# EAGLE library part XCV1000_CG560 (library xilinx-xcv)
xcv1000_cg560_1532 edit this description Auto generated by make-symbol-device-package-bsdl.ulp Rev. 26 Source: xcv1000_cg560_1532.bsd
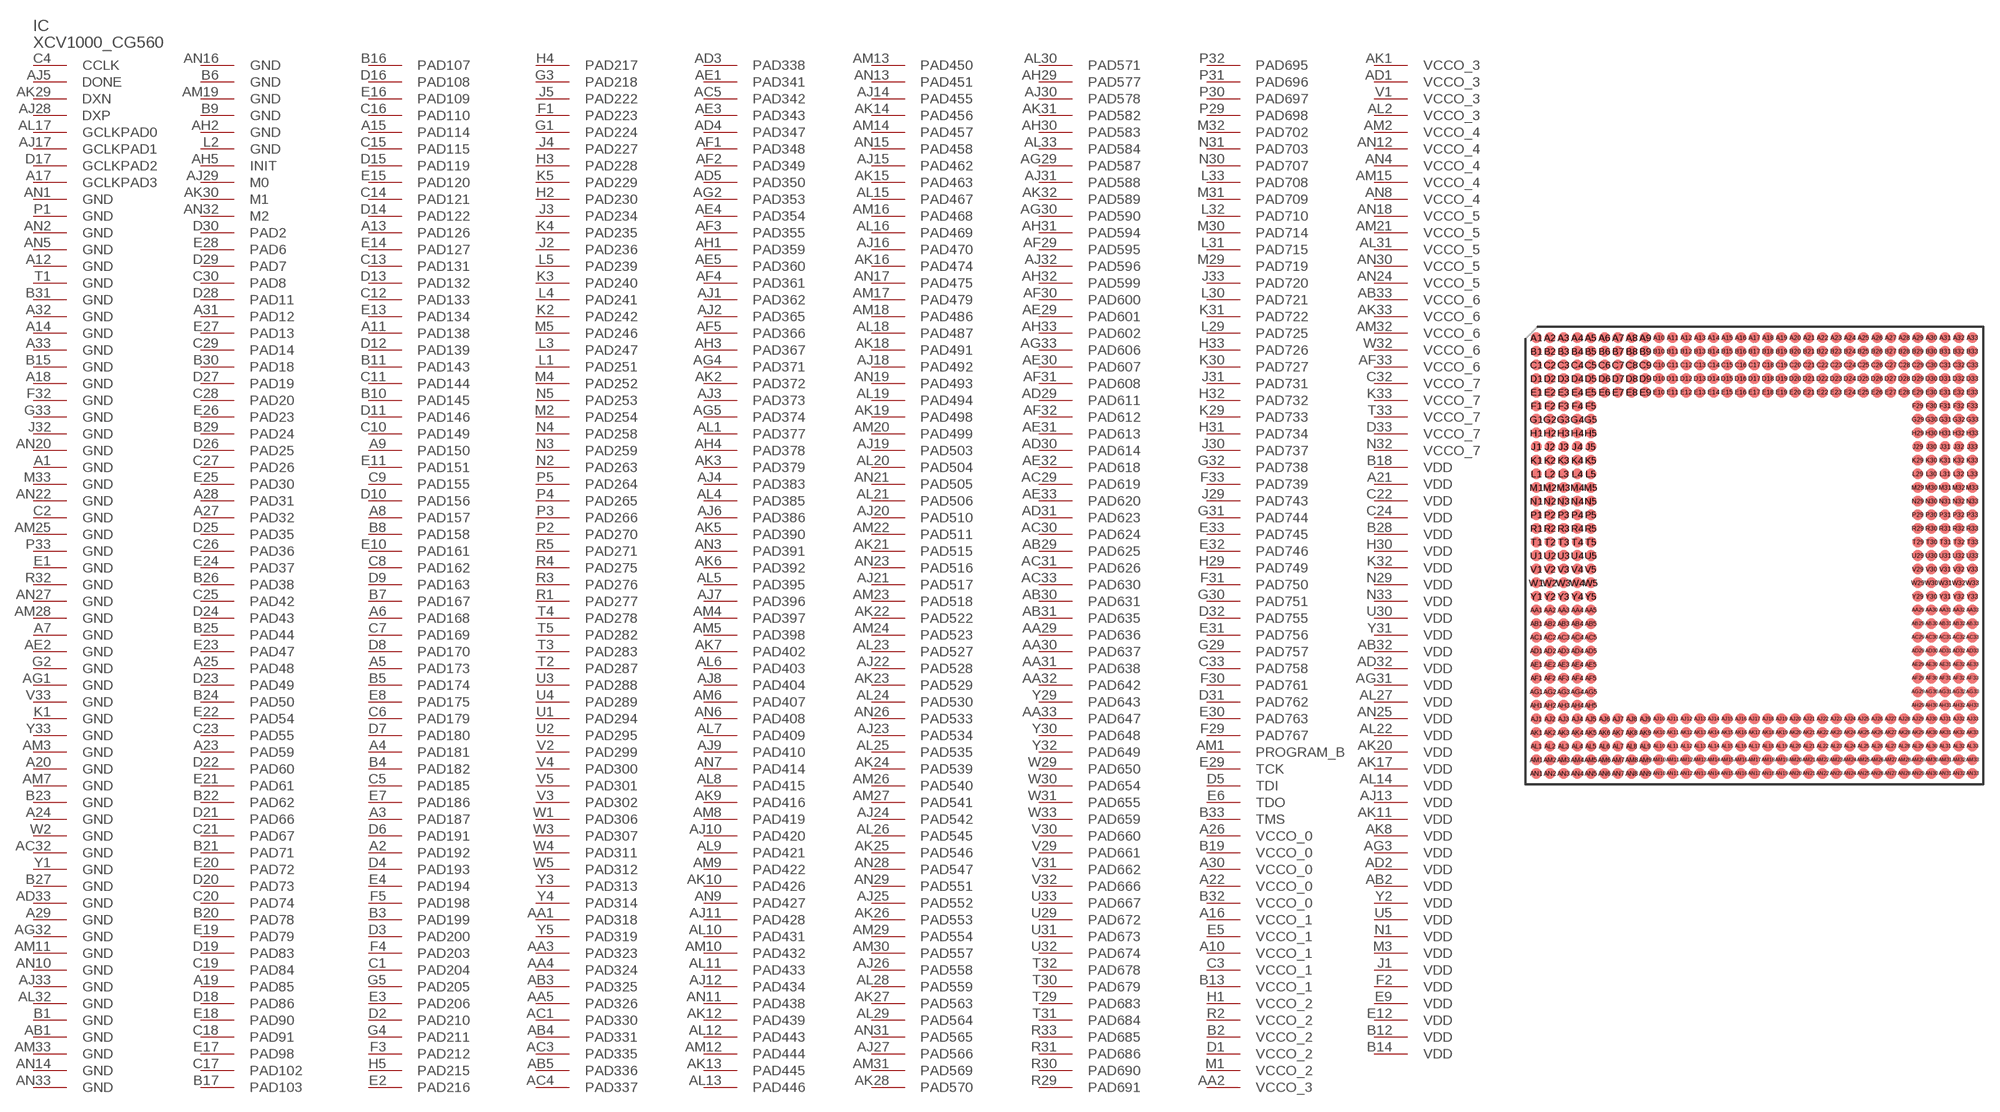
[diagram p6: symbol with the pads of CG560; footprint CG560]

Designator prefix IC

## XCV1000_CG560 (OC_FARNELL: unknown; OC_NEWARK: unknown)  [CG560]
A1  GND  pwr
A2  PAD192
A3  PAD187
A4  PAD181
A5  PAD173
A6  PAD168
A7  GND  pwr
A8  PAD157
A9  PAD150
A10  VCCO_1  pwr
A11  PAD138
A12  GND  pwr
A13  PAD126
A14  GND  pwr
A15  PAD114
A16  VCCO_1  pwr
A17  GCLKPAD3  in
A18  GND  pwr
A19  PAD85
A20  GND  pwr
A21  VDD  pwr
A22  VCCO_0  pwr
A23  PAD59
A24  GND  pwr
A25  PAD48
A26  VCCO_0  pwr
A27  PAD32
A28  PAD31
A29  GND  pwr
A30  VCCO_0  pwr
A31  PAD12
A32  GND  pwr
A33  GND  pwr
AA1  PAD318
AA2  VCCO_3  pwr
AA3  PAD323
AA4  PAD324
AA5  PAD326
AA29  PAD636
AA30  PAD637
AA31  PAD638
AA32  PAD642
AA33  PAD647
AB1  GND  pwr
AB2  VDD  pwr
AB3  PAD325
AB4  PAD331
AB5  PAD336
AB29  PAD625
AB30  PAD631
AB31  PAD635
AB32  VDD  pwr
AB33  VCCO_6  pwr
AC1  PAD330
AC3  PAD335
AC4  PAD337
AC5  PAD342
AC29  PAD619
AC30  PAD624
AC31  PAD626
AC32  GND  pwr
AC33  PAD630
AD1  VCCO_3  pwr
AD2  VDD  pwr
AD3  PAD338
AD4  PAD347
AD5  PAD350
AD29  PAD611
AD30  PAD614
AD31  PAD623
AD32  VDD  pwr
AD33  GND  pwr
AE1  PAD341
AE2  GND  pwr
AE3  PAD343
AE4  PAD354
AE5  PAD360
AE29  PAD601
AE30  PAD607
AE31  PAD613
AE32  PAD618
AE33  PAD620
AF1  PAD348
AF2  PAD349
AF3  PAD355
AF4  PAD361
AF5  PAD366
AF29  PAD595
AF30  PAD600
AF31  PAD608
AF32  PAD612
AF33  VCCO_6  pwr
AG1  GND  pwr
AG2  PAD353
AG3  VDD  pwr
AG4  PAD371
AG5  PAD374
AG29  PAD587
AG30  PAD590
AG31  VDD  pwr
AG32  GND  pwr
AG33  PAD606
AH1  PAD359
AH2  GND  pwr
AH3  PAD367
AH4  PAD378
AH5  INIT
AH29  PAD577
AH30  PAD583
AH31  PAD594
AH32  PAD599
AH33  PAD602
AJ1  PAD362
AJ2  PAD365
AJ3  PAD373
AJ4  PAD383
AJ5  DONE
AJ6  PAD386
AJ7  PAD396
AJ8  PAD404
AJ9  PAD410
AJ10  PAD420
AJ11  PAD428
AJ12  PAD434
AJ13  VDD  pwr
AJ14  PAD455
AJ15  PAD462
AJ16  PAD470
AJ17  GCLKPAD1  in
AJ18  PAD492
AJ19  PAD503
AJ20  PAD510
AJ21  PAD517
AJ22  PAD528
AJ23  PAD534
AJ24  PAD542
AJ25  PAD552
AJ26  PAD558
AJ27  PAD566
AJ28  DXP  pas
AJ29  M0  in
AJ30  PAD578
AJ31  PAD588
AJ32  PAD596
AJ33  GND  pwr
AK1  VCCO_3  pwr
AK2  PAD372
AK3  PAD379
AK5  PAD390
AK6  PAD392
AK7  PAD402
AK8  VDD  pwr
AK9  PAD416
AK10  PAD426
AK11  VDD  pwr
AK12  PAD439
AK13  PAD445
AK14  PAD456
AK15  PAD463
AK16  PAD474
AK17  VDD  pwr
AK18  PAD491
AK19  PAD498
AK20  VDD  pwr
AK21  PAD515
AK22  PAD522
AK23  PAD529
AK24  PAD539
AK25  PAD546
AK26  PAD553
AK27  PAD563
AK28  PAD570
AK29  DXN  pas
AK30  M1  in
AK31  PAD582
AK32  PAD589
AK33  VCCO_6  pwr
AL1  PAD377
AL2  VCCO_3  pwr
AL4  PAD385
AL5  PAD395
AL6  PAD403
AL7  PAD409
AL8  PAD415
AL9  PAD421
AL10  PAD431
AL11  PAD433
AL12  PAD443
AL13  PAD446
AL14  VDD  pwr
AL15  PAD467
AL16  PAD469
AL17  GCLKPAD0  in
AL18  PAD487
AL19  PAD494
AL20  PAD504
AL21  PAD506
AL22  VDD  pwr
AL23  PAD527
AL24  PAD530
AL25  PAD535
AL26  PAD545
AL27  VDD  pwr
AL28  PAD559
AL29  PAD564
AL30  PAD571
AL31  VCCO_5  pwr
AL32  GND  pwr
AL33  PAD584
AM1  PROGRAM_B  in
AM2  VCCO_4  pwr
AM3  GND  pwr
AM4  PAD397
AM5  PAD398
AM6  PAD407
AM7  GND  pwr
AM8  PAD419
AM9  PAD422
AM10  PAD432
AM11  GND  pwr
AM12  PAD444
AM13  PAD450
AM14  PAD457
AM15  VCCO_4  pwr
AM16  PAD468
AM17  PAD479
AM18  PAD486
AM19  GND  pwr
AM20  PAD499
AM21  VCCO_5  pwr
AM22  PAD511
AM23  PAD518
AM24  PAD523
AM25  GND  pwr
AM26  PAD540
AM27  PAD541
AM28  GND  pwr
AM29  PAD554
AM30  PAD557
AM31  PAD569
AM32  VCCO_6  pwr
AM33  GND  pwr
AN1  GND  pwr
AN2  GND  pwr
AN3  PAD391
AN4  VCCO_4  pwr
AN5  GND  pwr
AN6  PAD408
AN7  PAD414
AN8  VCCO_4  pwr
AN9  PAD427
AN10  GND  pwr
AN11  PAD438
AN12  VCCO_4  pwr
AN13  PAD451
AN14  GND  pwr
AN15  PAD458
AN16  GND  pwr
AN17  PAD475
AN18  VCCO_5  pwr
AN19  PAD493
AN20  GND  pwr
AN21  PAD505
AN22  GND  pwr
AN23  PAD516
AN24  VCCO_5  pwr
AN25  VDD  pwr
AN26  PAD533
AN27  GND  pwr
AN28  PAD547
AN29  PAD551
AN30  VCCO_5  pwr
AN31  PAD565
AN32  M2  in
AN33  GND  pwr
B1  GND  pwr
B2  VCCO_2  pwr
B3  PAD199
B4  PAD182
B5  PAD174
B6  GND  pwr
B7  PAD167
B8  PAD158
B9  GND  pwr
B10  PAD145
B11  PAD143
B12  VDD  pwr
B13  VCCO_1  pwr
B14  VDD  pwr
B15  GND  pwr
B16  PAD107
B17  PAD103
B18  VDD  pwr
B19  VCCO_0  pwr
B20  PAD78
B21  PAD71
B22  PAD62
B23  GND  pwr
B24  PAD50
B25  PAD44
B26  PAD38
B27  GND  pwr
B28  VDD  pwr
B29  PAD24
B30  PAD18
B31  GND  pwr
B32  VCCO_0  pwr
B33  TMS  in
C1  PAD204
C2  GND  pwr
C3  VCCO_1  pwr
C4  CCLK
C5  PAD185
C6  PAD179
C7  PAD169
C8  PAD162
C9  PAD155
C10  PAD149
C11  PAD144
C12  PAD133
C13  PAD131
C14  PAD121
C15  PAD115
C16  PAD110
C17  PAD102
C18  PAD91
C19  PAD84
C20  PAD74
C21  PAD67
C22  VDD  pwr
C23  PAD55
C24  VDD  pwr
C25  PAD42
C26  PAD36
C27  PAD26
C28  PAD20
C29  PAD14
C30  PAD8
C32  VCCO_7  pwr
C33  PAD758
D1  VCCO_2  pwr
D2  PAD210
D3  PAD200
D4  PAD193
D5  TDI  in
D6  PAD191
D7  PAD180
D8  PAD170
D9  PAD163
D10  PAD156
D11  PAD146
D12  PAD139
D13  PAD132
D14  PAD122
D15  PAD119
D16  PAD108
D17  GCLKPAD2  in
D18  PAD86
D19  PAD83
D20  PAD73
D21  PAD66
D22  PAD60
D23  PAD49
D24  PAD43
D25  PAD35
D26  PAD25
D27  PAD19
D28  PAD11
D29  PAD7
D30  PAD2
D31  PAD762
D32  PAD755
D33  VCCO_7  pwr
E1  GND  pwr
E2  PAD216
E3  PAD206
E4  PAD194
E5  VCCO_1  pwr
E6  TDO  out
E7  PAD186
E8  PAD175
E9  VDD  pwr
E10  PAD161
E11  PAD151
E12  VDD  pwr
E13  PAD134
E14  PAD127
E15  PAD120
E16  PAD109
E17  PAD98
E18  PAD90
E19  PAD79
E20  PAD72
E21  PAD61
E22  PAD54
E23  PAD47
E24  PAD37
E25  PAD30
E26  PAD23
E27  PAD13
E28  PAD6
E29  TCK  in
E30  PAD763
E31  PAD756
E32  PAD746
E33  PAD745
F1  PAD223
F2  VDD  pwr
F3  PAD212
F4  PAD203
F5  PAD198
F29  PAD767
F30  PAD761
F31  PAD750
F32  GND  pwr
F33  PAD739
G1  PAD224
G2  GND  pwr
G3  PAD218
G4  PAD211
G5  PAD205
G29  PAD757
G30  PAD751
G31  PAD744
G32  PAD738
G33  GND  pwr
H1  VCCO_2  pwr
H2  PAD230
H3  PAD228
H4  PAD217
H5  PAD215
H29  PAD749
H30  VDD  pwr
H31  PAD734
H32  PAD732
H33  PAD726
J1  VDD  pwr
J2  PAD236
J3  PAD234
J4  PAD227
J5  PAD222
J29  PAD743
J30  PAD737
J31  PAD731
J32  GND  pwr
J33  PAD720
K1  GND  pwr
K2  PAD242
K3  PAD240
K4  PAD235
K5  PAD229
K29  PAD733
K30  PAD727
K31  PAD722
K32  VDD  pwr
K33  VCCO_7  pwr
L1  PAD251
L2  GND  pwr
L3  PAD247
L4  PAD241
L5  PAD239
L29  PAD725
L30  PAD721
L31  PAD715
L32  PAD710
L33  PAD708
M1  VCCO_2  pwr
M2  PAD254
M3  VDD  pwr
M4  PAD252
M5  PAD246
M29  PAD719
M30  PAD714
M31  PAD709
M32  PAD702
M33  GND  pwr
N1  VDD  pwr
N2  PAD263
N3  PAD259
N4  PAD258
N5  PAD253
N29  VDD  pwr
N30  PAD707
N31  PAD703
N32  VCCO_7  pwr
N33  VDD  pwr
P1  GND  pwr
P2  PAD270
P3  PAD266
P4  PAD265
P5  PAD264
P29  PAD698
P30  PAD697
P31  PAD696
P32  PAD695
P33  GND  pwr
R1  PAD277
R2  VCCO_2  pwr
R3  PAD276
R4  PAD275
R5  PAD271
R29  PAD691
R30  PAD690
R31  PAD686
R32  GND  pwr
R33  PAD685
T1  GND  pwr
T2  PAD287
T3  PAD283
T4  PAD278
T5  PAD282
T29  PAD683
T30  PAD679
T31  PAD684
T32  PAD678
T33  VCCO_7  pwr
U1  PAD294
U2  PAD295
U3  PAD288
U4  PAD289
U5  VDD  pwr
U29  PAD672
U30  VDD  pwr
U31  PAD673
U32  PAD674
U33  PAD667
V1  VCCO_3  pwr
V2  PAD299
V3  PAD302
V4  PAD300
V5  PAD301
V29  PAD661
V30  PAD660
V31  PAD662
V32  PAD666
V33  GND  pwr
W1  PAD306
W2  GND  pwr
W3  PAD307
W4  PAD311
W5  PAD312
W29  PAD650
W30  PAD654
W31  PAD655
W32  VCCO_6  pwr
W33  PAD659
Y1  GND  pwr
Y2  VDD  pwr
Y3  PAD313
Y4  PAD314
Y5  PAD319
Y29  PAD643
Y30  PAD648
Y31  VDD  pwr
Y32  PAD649
Y33  GND  pwr

## Footprint CG560 (pad centres in mm)
xcv1000_cg560_1532 edit this description Auto generated by make-symbol-device-package-bsdl.ulp Rev. 26 Source: xcv1000_cg560_1532.bsd
smd 1 x 1: A1 -20.32,20.32; A2 -19.05,20.32; A3 -17.78,20.32; A4 -16.51,20.32; A5 -15.24,20.32; A6 -13.97,20.32; A7 -12.7,20.32; A8 -11.43,20.32; A9 -10.16,20.32; A10 -8.89,20.32; A11 -7.62,20.32; A12 -6.35,20.32; A13 -5.08,20.32; A14 -3.81,20.32; A15 -2.54,20.32; A16 -1.27,20.32; A17 0,20.32; A18 1.27,20.32; A19 2.54,20.32; A20 3.81,20.32; A21 5.08,20.32; A22 6.35,20.32; A23 7.62,20.32; A24 8.89,20.32; A25 10.16,20.32; A26 11.43,20.32; A27 12.7,20.32; A28 13.97,20.32; A29 15.24,20.32; A30 16.51,20.32; A31 17.78,20.32; A32 19.05,20.32; A33 20.32,20.32; AA1 -20.32,-5.08; AA2 -19.05,-5.08; AA3 -17.78,-5.08; AA4 -16.51,-5.08; AA5 -15.24,-5.08; AA29 15.24,-5.08; AA30 16.51,-5.08; AA31 17.78,-5.08; AA32 19.05,-5.08; AA33 20.32,-5.08; AB1 -20.32,-6.35; AB2 -19.05,-6.35; AB3 -17.78,-6.35; AB4 -16.51,-6.35; AB5 -15.24,-6.35; AB29 15.24,-6.35; AB30 16.51,-6.35; AB31 17.78,-6.35; AB32 19.05,-6.35; AB33 20.32,-6.35; AC1 -20.32,-7.62; AC2 -19.05,-7.62; AC3 -17.78,-7.62; AC4 -16.51,-7.62; AC5 -15.24,-7.62; AC29 15.24,-7.62; AC30 16.51,-7.62; AC31 17.78,-7.62; AC32 19.05,-7.62; AC33 20.32,-7.62; AD1 -20.32,-8.89; AD2 -19.05,-8.89; AD3 -17.78,-8.89; AD4 -16.51,-8.89; AD5 -15.24,-8.89; AD29 15.24,-8.89; AD30 16.51,-8.89; AD31 17.78,-8.89; AD32 19.05,-8.89; AD33 20.32,-8.89; AE1 -20.32,-10.16; AE2 -19.05,-10.16; AE3 -17.78,-10.16; AE4 -16.51,-10.16; AE5 -15.24,-10.16; AE29 15.24,-10.16; AE30 16.51,-10.16; AE31 17.78,-10.16; AE32 19.05,-10.16; AE33 20.32,-10.16; AF1 -20.32,-11.43; AF2 -19.05,-11.43; AF3 -17.78,-11.43; AF4 -16.51,-11.43; AF5 -15.24,-11.43; AF29 15.24,-11.43; AF30 16.51,-11.43; AF31 17.78,-11.43; AF32 19.05,-11.43; AF33 20.32,-11.43; AG1 -20.32,-12.7; AG2 -19.05,-12.7; AG3 -17.78,-12.7; AG4 -16.51,-12.7; AG5 -15.24,-12.7; AG29 15.24,-12.7; AG30 16.51,-12.7; AG31 17.78,-12.7; AG32 19.05,-12.7; AG33 20.32,-12.7; AH1 -20.32,-13.97; AH2 -19.05,-13.97; AH3 -17.78,-13.97; AH4 -16.51,-13.97; AH5 -15.24,-13.97; AH29 15.24,-13.97; AH30 16.51,-13.97; AH31 17.78,-13.97; AH32 19.05,-13.97; AH33 20.32,-13.97; AJ1 -20.32,-15.24; AJ2 -19.05,-15.24; AJ3 -17.78,-15.24; AJ4 -16.51,-15.24; AJ5 -15.24,-15.24; AJ6 -13.97,-15.24; AJ7 -12.7,-15.24; AJ8 -11.43,-15.24; AJ9 -10.16,-15.24; AJ10 -8.89,-15.24; AJ11 -7.62,-15.24; AJ12 -6.35,-15.24; AJ13 -5.08,-15.24; AJ14 -3.81,-15.24; AJ15 -2.54,-15.24; AJ16 -1.27,-15.24; AJ17 0,-15.24; AJ18 1.27,-15.24; AJ19 2.54,-15.24; AJ20 3.81,-15.24; AJ21 5.08,-15.24; AJ22 6.35,-15.24; AJ23 7.62,-15.24; AJ24 8.89,-15.24; AJ25 10.16,-15.24; AJ26 11.43,-15.24; AJ27 12.7,-15.24; AJ28 13.97,-15.24; AJ29 15.24,-15.24; AJ30 16.51,-15.24; AJ31 17.78,-15.24; AJ32 19.05,-15.24; AJ33 20.32,-15.24; AK1 -20.32,-16.51; AK2 -19.05,-16.51; AK3 -17.78,-16.51; AK4 -16.51,-16.51; AK5 -15.24,-16.51; AK6 -13.97,-16.51; AK7 -12.7,-16.51; AK8 -11.43,-16.51; AK9 -10.16,-16.51; AK10 -8.89,-16.51; AK11 -7.62,-16.51; AK12 -6.35,-16.51; AK13 -5.08,-16.51; AK14 -3.81,-16.51; AK15 -2.54,-16.51; AK16 -1.27,-16.51; AK17 0,-16.51; AK18 1.27,-16.51; AK19 2.54,-16.51; AK20 3.81,-16.51; AK21 5.08,-16.51; AK22 6.35,-16.51; AK23 7.62,-16.51; AK24 8.89,-16.51; AK25 10.16,-16.51; AK26 11.43,-16.51; AK27 12.7,-16.51; AK28 13.97,-16.51; AK29 15.24,-16.51; AK30 16.51,-16.51; AK31 17.78,-16.51; AK32 19.05,-16.51; AK33 20.32,-16.51; AL1 -20.32,-17.78; AL2 -19.05,-17.78; AL3 -17.78,-17.78; AL4 -16.51,-17.78; AL5 -15.24,-17.78; AL6 -13.97,-17.78; AL7 -12.7,-17.78; AL8 -11.43,-17.78; AL9 -10.16,-17.78; AL10 -8.89,-17.78; AL11 -7.62,-17.78; AL12 -6.35,-17.78; AL13 -5.08,-17.78; AL14 -3.81,-17.78; AL15 -2.54,-17.78; AL16 -1.27,-17.78; AL17 0,-17.78; AL18 1.27,-17.78; AL19 2.54,-17.78; AL20 3.81,-17.78; AL21 5.08,-17.78; AL22 6.35,-17.78; AL23 7.62,-17.78; AL24 8.89,-17.78; AL25 10.16,-17.78; AL26 11.43,-17.78; AL27 12.7,-17.78; AL28 13.97,-17.78; AL29 15.24,-17.78; AL30 16.51,-17.78; AL31 17.78,-17.78; AL32 19.05,-17.78; AL33 20.32,-17.78; AM1 -20.32,-19.05; AM2 -19.05,-19.05; AM3 -17.78,-19.05; AM4 -16.51,-19.05; AM5 -15.24,-19.05; AM6 -13.97,-19.05; AM7 -12.7,-19.05; AM8 -11.43,-19.05; AM9 -10.16,-19.05; AM10 -8.89,-19.05; AM11 -7.62,-19.05; AM12 -6.35,-19.05; AM13 -5.08,-19.05; AM14 -3.81,-19.05; AM15 -2.54,-19.05; AM16 -1.27,-19.05; AM17 0,-19.05; AM18 1.27,-19.05; AM19 2.54,-19.05; AM20 3.81,-19.05; AM21 5.08,-19.05; AM22 6.35,-19.05; AM23 7.62,-19.05; AM24 8.89,-19.05; AM25 10.16,-19.05; AM26 11.43,-19.05; AM27 12.7,-19.05; AM28 13.97,-19.05; AM29 15.24,-19.05; AM30 16.51,-19.05; AM31 17.78,-19.05; AM32 19.05,-19.05; AM33 20.32,-19.05; AN1 -20.32,-20.32; AN2 -19.05,-20.32; AN3 -17.78,-20.32; AN4 -16.51,-20.32; AN5 -15.24,-20.32; AN6 -13.97,-20.32; AN7 -12.7,-20.32; AN8 -11.43,-20.32; AN9 -10.16,-20.32; AN10 -8.89,-20.32; AN11 -7.62,-20.32; AN12 -6.35,-20.32; AN13 -5.08,-20.32; AN14 -3.81,-20.32; AN15 -2.54,-20.32; AN16 -1.27,-20.32; AN17 0,-20.32; AN18 1.27,-20.32; AN19 2.54,-20.32; AN20 3.81,-20.32; AN21 5.08,-20.32; AN22 6.35,-20.32; AN23 7.62,-20.32; AN24 8.89,-20.32; AN25 10.16,-20.32; AN26 11.43,-20.32; AN27 12.7,-20.32; AN28 13.97,-20.32; AN29 15.24,-20.32; AN30 16.51,-20.32; AN31 17.78,-20.32; AN32 19.05,-20.32; AN33 20.32,-20.32; B1 -20.32,19.05; B2 -19.05,19.05; B3 -17.78,19.05; B4 -16.51,19.05; B5 -15.24,19.05; B6 -13.97,19.05; B7 -12.7,19.05; B8 -11.43,19.05; B9 -10.16,19.05; B10 -8.89,19.05; B11 -7.62,19.05; B12 -6.35,19.05; B13 -5.08,19.05; B14 -3.81,19.05; B15 -2.54,19.05; B16 -1.27,19.05; B17 0,19.05; B18 1.27,19.05; B19 2.54,19.05; B20 3.81,19.05; B21 5.08,19.05; B22 6.35,19.05; B23 7.62,19.05; B24 8.89,19.05; B25 10.16,19.05; B26 11.43,19.05; B27 12.7,19.05; B28 13.97,19.05; B29 15.24,19.05; B30 16.51,19.05; B31 17.78,19.05; B32 19.05,19.05; B33 20.32,19.05; C1 -20.32,17.78; C2 -19.05,17.78; C3 -17.78,17.78; C4 -16.51,17.78; C5 -15.24,17.78; C6 -13.97,17.78; C7 -12.7,17.78; C8 -11.43,17.78; C9 -10.16,17.78; C10 -8.89,17.78; C11 -7.62,17.78; C12 -6.35,17.78; C13 -5.08,17.78; C14 -3.81,17.78; C15 -2.54,17.78; C16 -1.27,17.78; C17 0,17.78; C18 1.27,17.78; C19 2.54,17.78; C20 3.81,17.78; C21 5.08,17.78; C22 6.35,17.78; C23 7.62,17.78; C24 8.89,17.78; C25 10.16,17.78; C26 11.43,17.78; C27 12.7,17.78; C28 13.97,17.78; C29 15.24,17.78; C30 16.51,17.78; C31 17.78,17.78; C32 19.05,17.78; C33 20.32,17.78; D1 -20.32,16.51; D2 -19.05,16.51; D3 -17.78,16.51; D4 -16.51,16.51; D5 -15.24,16.51; D6 -13.97,16.51; D7 -12.7,16.51; D8 -11.43,16.51; D9 -10.16,16.51; D10 -8.89,16.51; D11 -7.62,16.51; D12 -6.35,16.51; D13 -5.08,16.51; D14 -3.81,16.51; D15 -2.54,16.51; D16 -1.27,16.51; D17 0,16.51; D18 1.27,16.51; D19 2.54,16.51; D20 3.81,16.51; D21 5.08,16.51; D22 6.35,16.51; D23 7.62,16.51; D24 8.89,16.51; D25 10.16,16.51; D26 11.43,16.51; D27 12.7,16.51; D28 13.97,16.51; D29 15.24,16.51; D30 16.51,16.51; D31 17.78,16.51; D32 19.05,16.51; D33 20.32,16.51; E1 -20.32,15.24; E2 -19.05,15.24; E3 -17.78,15.24; E4 -16.51,15.24; E5 -15.24,15.24; E6 -13.97,15.24; E7 -12.7,15.24; E8 -11.43,15.24; E9 -10.16,15.24; E10 -8.89,15.24; E11 -7.62,15.24; E12 -6.35,15.24; E13 -5.08,15.24; E14 -3.81,15.24; E15 -2.54,15.24; E16 -1.27,15.24; E17 0,15.24; E18 1.27,15.24; E19 2.54,15.24; E20 3.81,15.24; E21 5.08,15.24; E22 6.35,15.24; E23 7.62,15.24; E24 8.89,15.24; E25 10.16,15.24; E26 11.43,15.24; E27 12.7,15.24; E28 13.97,15.24; E29 15.24,15.24; E30 16.51,15.24; E31 17.78,15.24; E32 19.05,15.24; E33 20.32,15.24; F1 -20.32,13.97; F2 -19.05,13.97; F3 -17.78,13.97; F4 -16.51,13.97; F5 -15.24,13.97; F29 15.24,13.97; F30 16.51,13.97; F31 17.78,13.97; F32 19.05,13.97; F33 20.32,13.97; G1 -20.32,12.7; G2 -19.05,12.7; G3 -17.78,12.7; G4 -16.51,12.7; G5 -15.24,12.7; G29 15.24,12.7; G30 16.51,12.7; G31 17.78,12.7; G32 19.05,12.7; G33 20.32,12.7; H1 -20.32,11.43; H2 -19.05,11.43; H3 -17.78,11.43; H4 -16.51,11.43; H5 -15.24,11.43; H29 15.24,11.43; H30 16.51,11.43; H31 17.78,11.43; H32 19.05,11.43; H33 20.32,11.43; J1 -20.32,10.16; J2 -19.05,10.16; J3 -17.78,10.16; J4 -16.51,10.16; J5 -15.24,10.16; J29 15.24,10.16; J30 16.51,10.16; J31 17.78,10.16; J32 19.05,10.16; J33 20.32,10.16; K1 -20.32,8.89; K2 -19.05,8.89; K3 -17.78,8.89; K4 -16.51,8.89; K5 -15.24,8.89; K29 15.24,8.89; K30 16.51,8.89; K31 17.78,8.89; K32 19.05,8.89; K33 20.32,8.89; L1 -20.32,7.62; L2 -19.05,7.62; L3 -17.78,7.62; L4 -16.51,7.62; L5 -15.24,7.62; L29 15.24,7.62; L30 16.51,7.62; L31 17.78,7.62; L32 19.05,7.62; L33 20.32,7.62; M1 -20.32,6.35; M2 -19.05,6.35; M3 -17.78,6.35; M4 -16.51,6.35; M5 -15.24,6.35; M29 15.24,6.35; M30 16.51,6.35; M31 17.78,6.35; M32 19.05,6.35; M33 20.32,6.35; N1 -20.32,5.08; N2 -19.05,5.08; N3 -17.78,5.08; N4 -16.51,5.08; N5 -15.24,5.08; N29 15.24,5.08; N30 16.51,5.08; N31 17.78,5.08; N32 19.05,5.08; N33 20.32,5.08; P1 -20.32,3.81; P2 -19.05,3.81; P3 -17.78,3.81; P4 -16.51,3.81; P5 -15.24,3.81; P29 15.24,3.81; P30 16.51,3.81; P31 17.78,3.81; P32 19.05,3.81; P33 20.32,3.81; R1 -20.32,2.54; R2 -19.05,2.54; R3 -17.78,2.54; R4 -16.51,2.54; R5 -15.24,2.54; R29 15.24,2.54; R30 16.51,2.54; R31 17.78,2.54; R32 19.05,2.54; R33 20.32,2.54; T1 -20.32,1.27; T2 -19.05,1.27; T3 -17.78,1.27; T4 -16.51,1.27; T5 -15.24,1.27; T29 15.24,1.27; T30 16.51,1.27; T31 17.78,1.27; T32 19.05,1.27; T33 20.32,1.27; U1 -20.32,0; U2 -19.05,0; U3 -17.78,0; U4 -16.51,0; U5 -15.24,0; U29 15.24,0; U30 16.51,0; U31 17.78,0; U32 19.05,0; U33 20.32,0; V1 -20.32,-1.27; V2 -19.05,-1.27; V3 -17.78,-1.27; V4 -16.51,-1.27; V5 -15.24,-1.27; V29 15.24,-1.27; V30 16.51,-1.27; V31 17.78,-1.27; V32 19.05,-1.27; V33 20.32,-1.27; W1 -20.32,-2.54; W2 -19.05,-2.54; W3 -17.78,-2.54; W4 -16.51,-2.54; W5 -15.24,-2.54; W29 15.24,-2.54; W30 16.51,-2.54; W31 17.78,-2.54; W32 19.05,-2.54; W33 20.32,-2.54; Y1 -20.32,-3.81; Y2 -19.05,-3.81; Y3 -17.78,-3.81; Y4 -16.51,-3.81; Y5 -15.24,-3.81; Y29 15.24,-3.81; Y30 16.51,-3.81; Y31 17.78,-3.81; Y32 19.05,-3.81; Y33 20.32,-3.81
